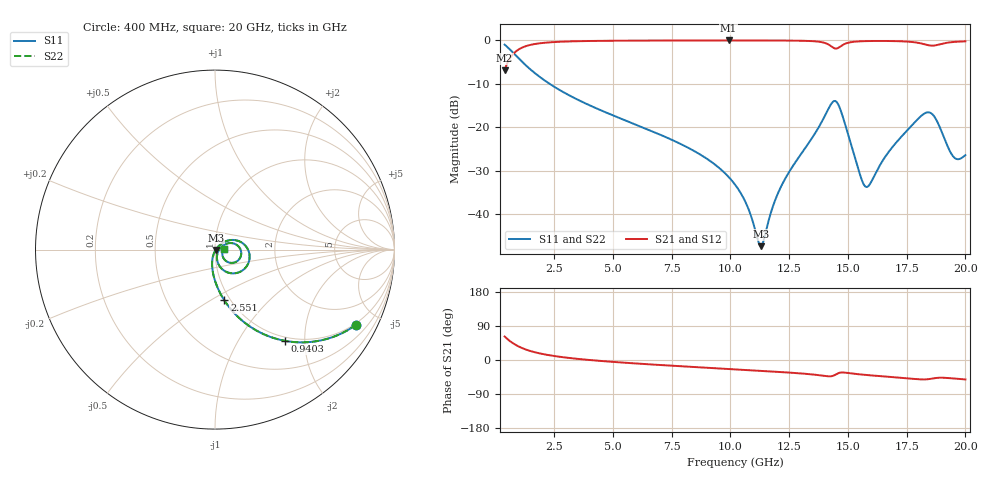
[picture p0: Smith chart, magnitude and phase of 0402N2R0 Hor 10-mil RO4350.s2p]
# GHz S MA R 50
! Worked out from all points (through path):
!   1960 points, 400 MHz to 20 GHz, reference 50 ohm
!   highest |S21| = -0.04 dB at 9.925 GHz (marker M1); lowest = -6.9 dB at 400 MHz (marker M2)
!   group delay of S21, straight-line fit = 11.1 ps
!   lowest |S11| = -47.4 dB at 11.3 GHz (marker M3), VSWR 1.01, Z = 50.4 - j0.23 ohm
!   |S11| at or under -10 dB: 2.31 GHz to end of sweep
!   |S22| runs from -47.4 to -1.0 dB; largest |S21 - S12| = 0
!   S11 on the Smith chart (normalised r, x): 400 MHz: 0.93, -3.81; 940.3 MHz: 0.93, -1.62; 2.551 GHz: 0.94, -0.58; 20 GHz: 1.10, +0.01
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0.4  0.8919 -27.9  0.4519 62.1  0.4519 62.1  0.8919 -27.9
0.9402757  0.6415 -52.5  0.7664 37.5  0.7664 37.5  0.6415 -52.5
1.580602  0.4427 -67.7  0.8956 22.2  0.8956 22.2  0.4427 -67.7
2.551097  0.2875 -79.6  0.9563 10.2  0.9563 10.2  0.2875 -79.6
3.671669  0.1974 -87.5  0.9785 2.0  0.9785 2.0  0.1974 -87.5
6.943338  0.08368 -101.3  0.9937 -12.9  0.9937 -12.9  0.08368 -101.3
8.764267  0.04769 -106.1  0.9956 -19.6  0.9956 -19.6  0.04769 -106.1
9.92486  0.02684 -106.5  0.9959 -23.7  0.9959 -23.7  0.02684 -106.5
10.205  0.02178 -105.5  0.9959 -24.6  0.9959 -24.6  0.02178 -105.5
10.71526  0.0125 -98.9  0.9957 -26.5  0.9957 -26.5  0.0125 -98.9
11.29556  0.004276 -32.3  0.9953 -28.5  0.9953 -28.5  0.004276 -32.3
12.13599  0.02013 42.0  0.9936 -31.7  0.9936 -31.7  0.02013 42.0
13.46667  0.07435 38.2  0.979 -38.0  0.979 -38.0  0.07435 38.2
14.09699  0.148 17.1  0.9167 -42.7  0.9167 -42.7  0.148 17.1
14.45717  0.2004 -23.9  0.8047 -39.2  0.8047 -39.2  0.2004 -23.9
14.93742  0.09666 -74.4  0.9241 -33.7  0.9241 -33.7  0.09666 -74.4
15.73783  0.02085 -34.4  0.9786 -39.3  0.9786 -39.3  0.02085 -34.4
16.73834  0.05205 27.1  0.9816 -44.3  0.9816 -44.3  0.05205 27.1
18.41919  0.1485 -12.6  0.878 -50.6  0.878 -50.6  0.1485 -12.6
18.74936  0.1235 -36.7  0.8777 -47.4  0.8777 -47.4  0.1235 -36.7
19.48974  0.04578 -28.0  0.9563 -48.7  0.9563 -48.7  0.04578 -28.0
20  0.04772 6.6  0.973 -51.2  0.973 -51.2  0.04772 6.6
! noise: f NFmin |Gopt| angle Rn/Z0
0.4  0.001271  0.7974  4.104  0.001297
2.571  0.005067  0.6794  7.907  0.003042
4.752  0.008075  0.6381  13.06  0.004156
6.933  0.01085  0.615  18.3  0.005114
9.104  0.01373  0.6064  23.46  0.0062
11.29  0.01797  0.6271  28.53  0.008507
13.47  0.03945  0.7812  33.68  0.03392
15.64  0.04758  0.7915  38.96  0.04191
17.82  0.07034  0.838  43.91  0.07913
20  0.05604  0.7827  48.85  0.04402
